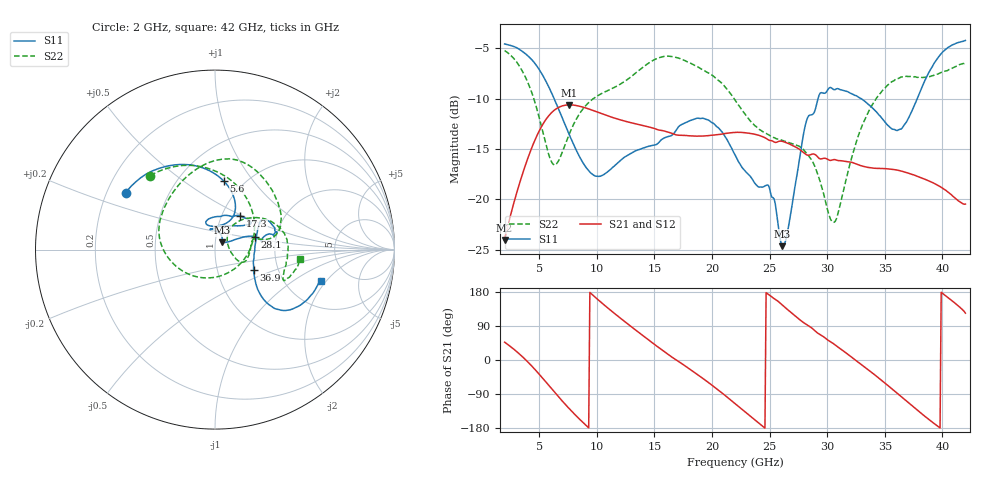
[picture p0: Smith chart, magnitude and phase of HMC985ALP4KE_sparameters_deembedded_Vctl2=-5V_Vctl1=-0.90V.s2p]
!s2p File: Measurements: S11, S21, S12, S22
# GHz S dB R 50.0
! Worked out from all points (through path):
!   401 points, 2 GHz to 42 GHz, reference 50 ohm
!   highest |S21| = -10.63 dB at 7.6 GHz (marker M1); lowest = -24.1 dB at 2 GHz (marker M2)
!   lowest |S11| = -24.7 dB at 26.1 GHz (marker M3), VSWR 1.12, Z = 54.1 + j4.51 ohm
!   |S11| at or under -10 dB: 6.296 GHz to 29.21 GHz (22.91 GHz wide, 129 % of centre); 32.94 GHz to 37.82 GHz (4.886 GHz wide, 13.8 % of centre)
!   |S22| runs from -22.3 to -5.2 dB; largest |S21 - S12| = 0.00033
!   S11 on the Smith chart (normalised r, x): 2 GHz: 0.28, +0.27; 5.6 GHz: 0.81, +0.73; 17.3 GHz: 1.22, +0.48; 28.1 GHz: 1.55, +0.23; 36.9 GHz: 1.50, -0.36; 42 GHz: 3.14, -1.74
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2  -4.57 147.6  -24.06 47.0  -24.07 47.0  -5.23 131.2
3.6  -5.37 121.0  -17.33 7.1  -17.33 7.1  -7.40 86.3
4.7  -6.62 100.1  -13.95 -27.2  -13.96 -27.2  -10.63 44.5
5.6  -8.31 82.5  -12.06 -58.6  -12.06 -58.6  -14.62 -6.1
6.4  -10.28 69.7  -11.08 -87.2  -11.09 -87.2  -16.58 -70.5
7.6  -13.55 61.3  -10.63 -128.0  -10.63 -128.0  -13.55 -142.9
8.7  -16.19 68.4  -10.82 -161.9  -10.82 -161.9  -11.18 -174.9
12  -16.21 109.0  -12.10 111.6  -12.11 111.6  -8.60 137.4
15.4  -14.35 78.4  -13.13 32.5  -13.13 32.5  -5.95 86.0
17.3  -12.62 53.3  -13.65 -7.9  -13.65 -7.9  -6.06 63.5
19.7  -12.14 35.9  -13.68 -59.6  -13.69 -59.6  -7.46 30.9
22  -15.59 52.9  -13.36 -115.0  -13.37 -115.0  -10.13 11.3
24.9  -18.63 98.2  -14.10 173.1  -14.11 173.1  -13.60 11.7
26.1  -24.67 45.4  -14.25 145.2  -14.26 145.3  -14.15 -1.4
28.1  -12.67 18.0  -15.51 95.7  -15.52 95.7  -15.29 -23.7
28.7  -11.60 10.5  -15.52 83.6  -15.53 83.6  -16.18 -25.7
30.6  -9.12 17.1  -16.06 41.7  -16.07 41.7  -22.29 19.7
33  -10.04 32.1  -16.69 -13.0  -16.70 -12.9  -12.79 47.2
35.4  -12.79 9.8  -17.00 -70.5  -17.00 -70.5  -8.54 20.4
36.9  -12.29 -27.8  -17.36 -108.8  -17.37 -108.7  -7.79 2.6
39.6  -5.99 -42.4  -18.61 -174.7  -18.62 -174.7  -7.57 -24.0
42  -4.23 -16.3  -20.48 123.6  -20.49 123.6  -6.41 -6.1
